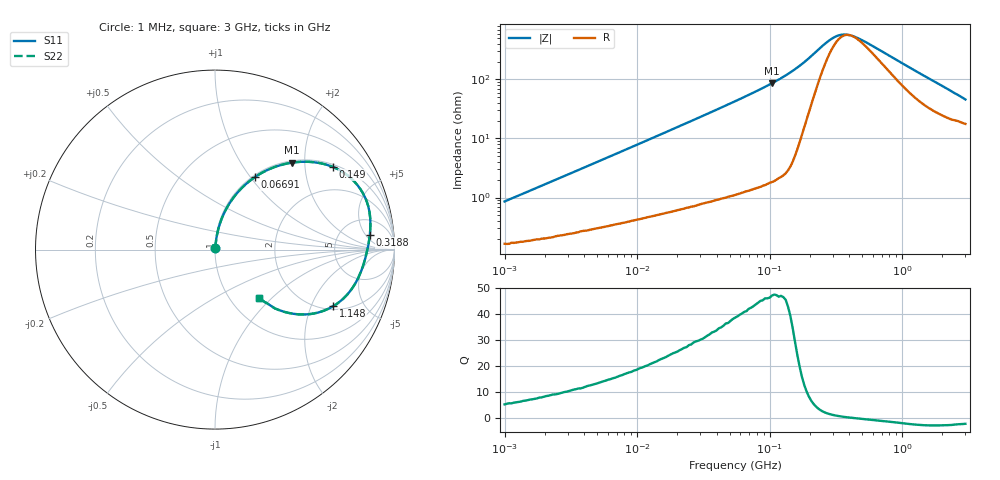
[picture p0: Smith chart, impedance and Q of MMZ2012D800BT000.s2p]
! S-parameter Generated by TDK Corporation
! Copyright(C) 2016 TDK Corporation.
! All Rights Reserved.
! TDK P/N: MMZ2012D800BT000 (Chip Beads)
! Property: |Z|=80¶ at 100MHz
! Size(LxWxT): 2x1.25x0.85mm, 0.079x0.049x0.033inches
! Model Type: s2p (Touchstone File Format Version 1.0)
! Frequency: DC=Yes Start=1MHz Stop=3000MHz 202points Log-sweep
! Note: This model was converted from impedance.
! Model Generated on May. 16, 2016
! Hash(MD5):
! Port Assignments:
!  1 ---@@@--- 2
! Applicable Conditions:
!  Temperature = 25 degC
!  DC Bias Current = 0 A
!  Small Signal Operation
! Terms and conditions regarding TDK Simulation Models
! (1)This simulation model is being provided solely for informational purposes. Please refer to the specifications of the products in terms of detailed characteristics of such products.
! (2)In no event shall TDK Corporation of any of its subsidiaries be liable for any loss or damage arising, directly or indirectly,
!  From any information contained in this simulation model, including, but not limited to loss or damages arising from any inaccuracies, omissions or errors in connection with such information.
! (3)Any and all copyrights on this simulation model are owned by TDK Corporation.
!  Duplication or redistribution of this simulation model without prior written permission from TDK Corporation is prohibited.
! (4)This simulation model is subject to any modification or change without any prior notice.
! (5)Neither TDK Corporation nor any of its subsidiaries shall make any warranty, express or implied,
!  Including but not limited to the correctness, implied warranties of merchantability and fitness for a particular purpose with respect to this simulation models.
! (6)The use of this simulation model shall be deemed to have consented to the terms and conditions hereof.
# MHz S MA R 50
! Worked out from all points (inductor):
!   201 points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, 1 MHz to 3 GHz, reference 50 ohm
!   read as one part in series: L = 133 nH near 1.041 MHz
!   highest Q = 47.2 at 103.9 MHz (marker M1), where L = 132 nH
!   self-resonance near 402.9 MHz
!   S11 on the Smith chart (normalised r, x): 1 MHz: 1.00, +0.02; 66.91 MHz: 1.03, +1.05; 149 MHz: 1.08, +2.79; 318.8 MHz: 10, +6; 1.148 GHz: 2.17, -2.93; 3 GHz: 1.35, -0.85
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1  0.008557 78.5  0.9983 -0.5  0.9983 -0.5  0.008557 78.5
3.900413  0.03142 83.3  0.9968 -1.8  0.9968 -1.8  0.03142 83.3
8.017732  0.06298 83.0  0.9943 -3.6  0.9943 -3.6  0.06298 83.0
14.61624  0.1126 81.0  0.9886 -6.5  0.9886 -6.5  0.1126 81.0
31.27247  0.2331 74.7  0.9648 -13.5  0.9648 -13.5  0.2331 74.7
54.77226  0.3888 65.6  0.9113 -22.9  0.9113 -22.9  0.3888 65.6
66.90963  0.4611 61.2  0.8762 -27.5  0.8762 -27.5  0.4611 61.2
103.9275  0.6457 48.6  0.7501 -40.2  0.7501 -40.2  0.6457 48.6
126.9575  0.7348 41.5  0.6627 -47.3  0.6627 -47.3  0.7348 41.5
149.005  0.8023 35.0  0.5743 -53.3  0.5743 -53.3  0.8023 35.0
182.0241  0.8637 26.1  0.4411 -59.4  0.4411 -59.4  0.8637 26.1
213.6344  0.8855 19.0  0.3307 -60.5  0.3307 -60.5  0.8855 19.0
271.6345  0.8793 10.0  0.2036 -48.8  0.2036 -48.8  0.8793 10.0
318.8066  0.8669 5.5  0.1602 -31.1  0.1602 -31.1  0.8669 5.5
374.1707  0.8547 1.6  0.1476 -9.5  0.1476 -9.5  0.8547 1.6
439.1493  0.8434 -1.9  0.1594 9.8  0.1594 9.8  0.8434 -1.9
800.5644  0.7957 -15.4  0.315 42.3  0.315 42.3  0.7957 -15.4
1147.801  0.7308 -25.5  0.4636 42.7  0.4636 42.7  0.7308 -25.5
1459.42  0.6591 -32.6  0.5691 38.6  0.5691 38.6  0.6591 -32.6
1782.824  0.5845 -38.1  0.6489 33.7  0.6489 33.7  0.5845 -38.1
2266.846  0.4852 -43.6  0.7301 27.3  0.7301 27.3  0.4852 -43.6
3000  0.3664 -47.6  0.7998 19.8  0.7998 19.8  0.3664 -47.6
